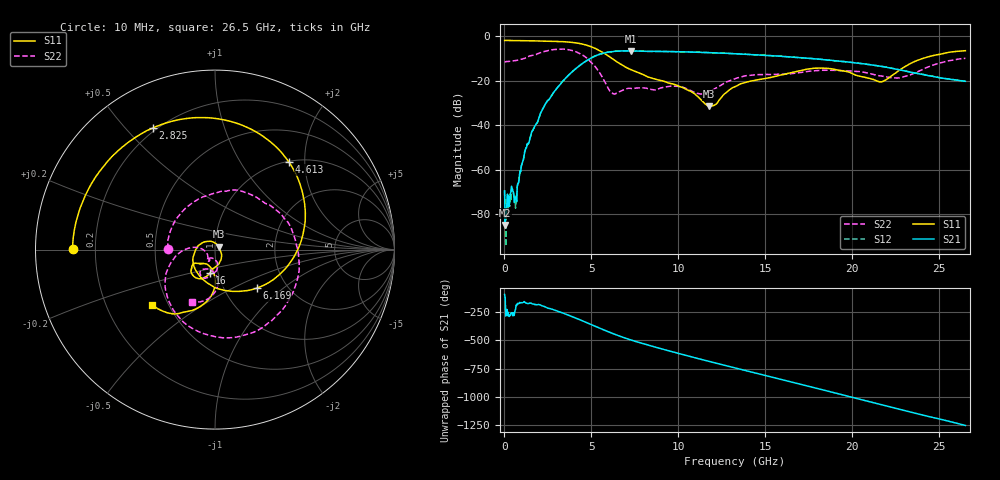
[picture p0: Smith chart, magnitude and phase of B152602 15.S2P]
!  2-Port S-parameters saved by WinCal
! VAR MeasName=S-Parameters (CALIBRATED_DATA) read from VNA (N5242A)
! VAR MeasDate=2016-1-5 16:27:27
! VAR NAME=B152602 15
! VAR FILENAME=B152602 15.S2P
! VAR DATE=2016-1-5 16:27:27
! VAR PHYS_PORTS=1,2
# Hz S DB R 50
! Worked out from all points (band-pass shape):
!   801 points, 10 MHz to 26.5 GHz, reference 50 ohm
!   highest |S21| = -6.68 dB at 7.295 GHz (marker M1); lowest = -84.8 dB at 43.11 MHz (marker M2)
!   |S21| within 3 dB of the highest: 5.032 GHz to 16.92 GHz (11.89 GHz wide, 108 % of centre)
!   lowest |S11| = -31.6 dB at 11.76 GHz (marker M3), VSWR 1.05, Z = 52.1 + j1.64 ohm
!   |S11| at or under -10 dB: 6.169 GHz to 24.09 GHz (17.92 GHz wide, 118 % of centre)
!   |S22| runs from -26.1 to -5.9 dB; largest |S21 - S12| = 0.0025
!   S11 on the Smith chart (normalised r, x): 10 MHz: 0.12, +0.00; 2.825 GHz: 0.18, +0.60; 4.613 GHz: 1.01, +1.67; 6.169 GHz: 1.41, -0.68; 16 GHz: 0.91, -0.24; 26.5 GHz: 0.41, -0.32
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1e7  -2.02 179.7  -69.56 -94.4  -69.53 63.2  -11.61 179.2
4.31125e7  -2.01 179.1  -84.81 -122.7  -83.36 -33.4  -11.59 176.8
1.755625e8  -2.02 176.4  -71.02 79.5  -71.96 84.5  -11.46 165.8
6.7225e8  -2.07 166.2  -72.36 172.9  -73.61 168.1  -10.97 125.7
1.46695e9  -2.17 149.7  -46.04 -172.0  -46.05 -172.4  -8.95 66.3
2.824562e9  -2.36 117.1  -25.37 131.2  -25.37 131.1  -6.10 -27.9
3.619262e9  -2.68 92.1  -18.11 86.6  -18.13 86.5  -6.05 -80.5
4.447075e9  -3.57 58.0  -12.56 35.6  -12.57 35.7  -8.38 -133.1
4.612638e9  -3.89 50.0  -11.63 25.1  -11.65 25.3  -9.17 -142.9
5.407338e9  -6.31 6.1  -8.38 -27.4  -8.38 -27.2  -15.74 179.3
6.168925e9  -10.00 -42.8  -7.04 -75.9  -7.04 -75.8  -25.51 -163.1
7.29475e9  -15.24 -117.3  -6.68 -137.6  -6.68 -137.5  -23.57 -129.2
8.851038e9  -19.77 175.9  -6.90 152.5  -6.89 152.4  -23.78 -117.2
1.027488e10  -23.27 139.7  -7.11 93.7  -7.12 93.7  -23.03 -124.5
1.176494e10  -31.63 36.9  -7.48 34.0  -7.46 34.1  -25.17 -90.3
1.3255e10  -22.74 -67.9  -7.96 -23.7  -7.95 -23.7  -19.16 -84.0
1.600334e10  -17.38 -102.8  -9.20 -129.6  -9.15 -129.6  -17.24 -103.4
1.769208e10  -14.58 -119.9  -10.16 165.6  -10.13 165.7  -15.72 -106.1
1.964571e10  -15.87 -143.5  -11.60 90.3  -11.58 90.1  -15.67 -118.2
2.209604e10  -18.80 -97.3  -14.25 -7.1  -14.21 -7.3  -18.59 -114.7
2.388411e10  -10.50 -99.9  -17.06 -74.6  -17.00 -74.9  -15.60 -84.7
2.65e10  -6.61 -138.5  -20.36 -172.8  -20.35 -173.2  -10.02 -113.5
